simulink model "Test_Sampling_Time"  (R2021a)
settings: Solver=FixedStepDiscrete  StartTime=0.0  StopTime=Inf  RelTol=1e-3  EnableMultiTasking=on
undefined symbols (not defined in the file): ADCINA0, ADCINA1, ADCINA2, ADCINA3, ADCINA4, ADCINA5, ADCINA6, ADCINA7, ADCINB0, ADCINB1, ADCINB2, ADCINB3, ADCINB4, ADCINB5, ADCINB6, ADCINB7
libraries: c2833xlib x3, c280xlib x1, dspstat3 x1, spsRMSLib x1

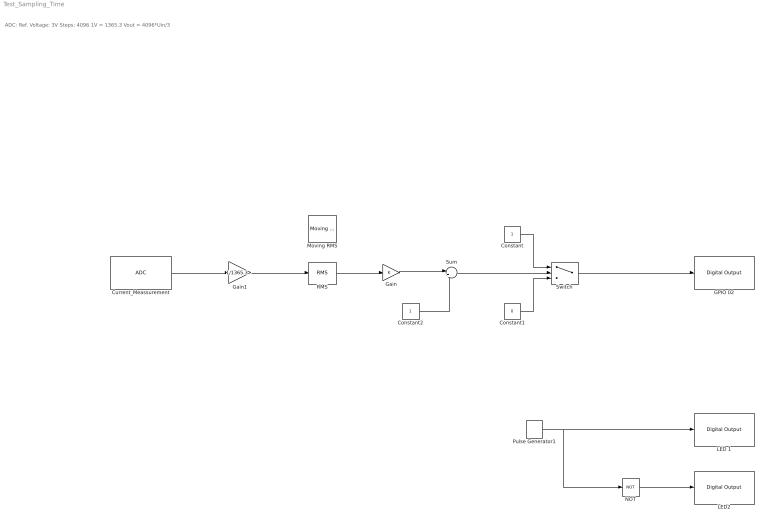
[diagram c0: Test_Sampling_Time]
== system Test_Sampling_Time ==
  note: ADC: Ref. Voltage: 3V Steps: 4096 1V = 1365.3 Vout = 4096*Uin/3
  Constant : Constant
  Constant1 : Constant  Value=0
  Constant2 : Constant
  Current_Meassurement : c280xlib/ADC  useModule=A  useMode=Sequential  sourceSOC=Software  sourceSOC1=Software  sourceSOC2=ePWMxB  xint2_ADCSOC=31  Ts=2e-6  dType=double  postInterrupt=off  numConversionsSingle=1  numConversionsDouble=1  conv0=ADCINA0  conv1=ADCINA1  conv2=ADCINA2  conv3=ADCINA3  conv4=ADCINA4  conv5=ADCINA5  conv6=ADCINA6  conv7=ADCINA7  conv8=ADCINB0  conv9=ADCINB1  conv10=ADCINB2  conv11=ADCINB3  conv12=ADCINB4  conv13=ADCINB5  conv14=ADCINB6  conv15=ADCINB7  convAB0=ADCINA0 and ADCINB0  convAB1=ADCINA1 and ADCINB1  convAB2=ADCINA2 and ADCINB2  convAB3=ADCINA3 and ADCINB3  convAB4=ADCINA4 and ADCINB4  convAB5=ADCINA5 and ADCINB5  convAB6=ADCINA6 and ADCINB6  convAB7=ADCINA7 and ADCINB7  convA0=ADCINA0  convA1=ADCINA1  convA2=ADCINA2  convA3=ADCINA3  convA4=ADCINA4  convA5=ADCINA5  convA6=ADCINA6  convA7=ADCINA7  convB0=ADCINB0  convB1=ADCINB1  convB2=ADCINB2  convB3=ADCINB3  convB4=ADCINB4  convB5=ADCINB5  convB6=ADCINB6  convB7=ADCINB7  c28xmultiPort=off  endma=off  chdma=1
  GPIO 02 : c2833xlib/Digital Output  GPIO_Number=GPIO0~GPIO7  GPIO_Bit0=off  GPIO_BIT0_Toggle=off  GPIO_Bit1=off  GPIO_BIT1_Toggle=off  GPIO_Bit2=on  GPIO_BIT2_Toggle=off  GPIO_Bit3=off  GPIO_BIT3_Toggle=off  GPIO_Bit4=off  GPIO_BIT4_Toggle=off  GPIO_Bit5=off  GPIO_BIT5_Toggle=off  GPIO_Bit6=off  GPIO_BIT6_Toggle=off  GPIO_Bit7=off  GPIO_BIT7_Toggle=off
  Gain : Gain
  Gain1 : Gain  Gain=1/1365.3
  LED 1 : c2833xlib/Digital Output  GPIO_Number=GPIO24~GPIO31  GPIO_Bit0=off  GPIO_BIT0_Toggle=off  GPIO_Bit1=off  GPIO_BIT1_Toggle=off  GPIO_Bit2=off  GPIO_BIT2_Toggle=off  GPIO_Bit3=off  GPIO_BIT3_Toggle=off  GPIO_Bit4=off  GPIO_BIT4_Toggle=off  GPIO_Bit5=off  GPIO_BIT5_Toggle=off  GPIO_Bit6=off  GPIO_BIT6_Toggle=off  GPIO_Bit7=on  GPIO_BIT7_Toggle=off
  LED2 : c2833xlib/Digital Output  GPIO_Number=GPIO32~GPIO39  GPIO_Bit0=off  GPIO_BIT0_Toggle=off  GPIO_Bit1=off  GPIO_BIT1_Toggle=off  GPIO_Bit2=on  GPIO_BIT2_Toggle=off  GPIO_Bit3=off  GPIO_BIT3_Toggle=off  GPIO_Bit4=off  GPIO_BIT4_Toggle=off  GPIO_Bit5=off  GPIO_BIT5_Toggle=off  GPIO_Bit6=off  GPIO_BIT6_Toggle=off  GPIO_Bit7=off  GPIO_BIT7_Toggle=off
  Moving RMS : dspstat3/Moving RMS  Commented=on  Method=Sliding window  ForgettingFactorPort=off  SpecifyWindowLength=on  WindowLength=1000  ForgettingFactor=0  SimulateUsing=Code generation
  NOT : Logic  Operator=NOT  IconShape=distinctive  AllPortsSameDT=off  OutDataTypeStr=boolean
  Pulse Generator1 : DiscretePulseGenerator  PulseType=Time based  PulseWidth=50
  RMS : spsRMSLib/RMS  Commented=through  TrueRMS=on  Freq=50  RMSInit=0  Ts=200e-6
  Sum : Sum  Inputs=|+-
  Switch : Switch  Criteria=u2 > Threshold
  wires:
  Gain1/1 -> RMS/1
  Switch/1 -> GPIO 02/1
  RMS/1 -> Gain/1
  Constant2/1 -> Sum/2
  Sum/1 -> Switch/2
  Constant/1 -> Switch/1
  Constant1/1 -> Switch/3
  Current_Meassurement/1 -> Gain1/1
  Gain/1 -> Sum/1
  Pulse Generator1/1 -> NOT/1, LED 1/1
  NOT/1 -> LED2/1
